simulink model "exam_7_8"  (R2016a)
settings: Solver=VariableStepAuto  StartTime=0.0  StopTime=10.0  RelTol=1e-3

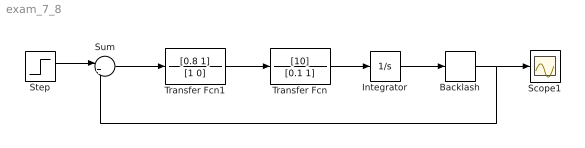
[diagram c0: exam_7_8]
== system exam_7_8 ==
  Backlash : Backlash
  Integrator : Integrator  InitialCondition=0.2
  Scope1 : Scope
  Step : Step  SampleTime=0
  Sum : Sum  Inputs=|+-
  Transfer Fcn : TransferFcn  Numerator=[10]  Denominator=[0.1 1]
  Transfer Fcn1 : TransferFcn  Numerator=[0.8 1]  Denominator=[1 0]
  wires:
  Sum/1 -> Transfer Fcn1/1
  Transfer Fcn/1 -> Integrator/1
  Transfer Fcn1/1 -> Transfer Fcn/1
  Step/1 -> Sum/1
  Integrator/1 -> Backlash/1
  Backlash/1 -> Sum/2, Scope1/1
